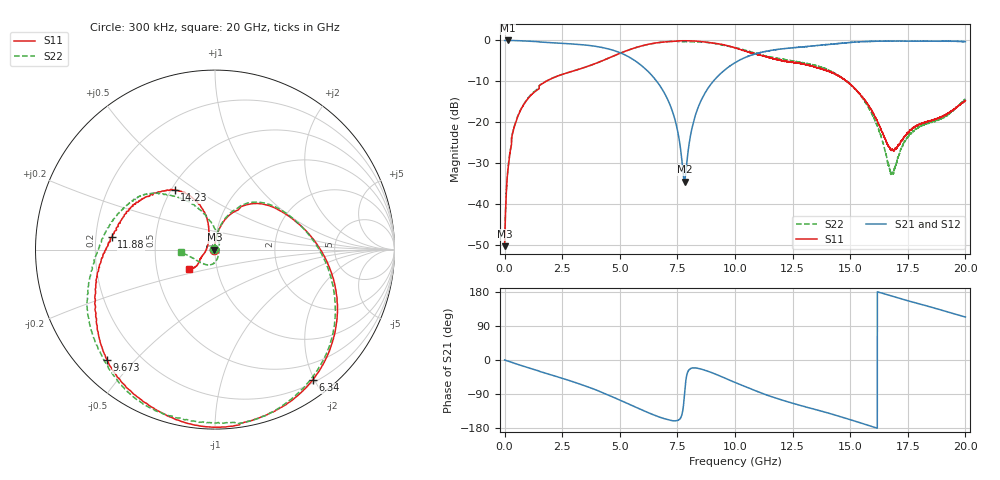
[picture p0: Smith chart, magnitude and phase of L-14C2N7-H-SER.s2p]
!{L-14C2N7}
!Johanson Technology Inc.
!www.johansontechnology.com
!Test Board Conditions:
!Substrate Type  RO4350B
!Substrate Thickness  20 mil
!Substrate Dk  3.66
!TL Type: GCPW
!TL Trace Width  36 mil
!TL Gap  12 mil
!Electrode orientation  Horizontal
!DUT TOPOLOGY	SERIES
!Mounting Pad LxW  26x36 mil
! Created Sun Jun 20 12:55:36 2021
# hz S ma R 50
! 2 Port Network Data from SP1.SP block
! freq  magS11  angS11  magS21  angS21  magS12  angS12  magS22  angS22
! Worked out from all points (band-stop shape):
!   20001 points, 300 kHz to 20 GHz, reference 50 ohm
!   highest |S21| = -0.02 dB at 130.3 MHz (marker M1); lowest = -34.6 dB at 7.81 GHz (marker M2)
!   |S21| within 3 dB of the highest: start of sweep to 5.007 GHz; 11.08 GHz to end of sweep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
!   lowest |S11| = -50.4 dB at 300 kHz (marker M3), VSWR 1.01, Z = 49.7 + j0.0289 ohm
!   |S11| at or under -10 dB: start of sweep to 1.807 GHz; 1.807622 GHz to 1.808451 GHz (828.7 kHz wide, 0.0458 % of centre); 14.85 GHz to end of sweep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
!   |S22| runs from -50.1 to -0.2 dB; largest |S21 - S12| = 0.016
!   S11 on the Smith chart (normalised r, x): 300 kHz: 0.99, +0.00; 6.34 GHz: 0.24, -1.97; 9.673 GHz: 0.09, -0.42; 11.88 GHz: 0.27, +0.06; 14.23 GHz: 0.52, +0.41; 20 GHz: 0.73, -0.17
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300000  0.003034 174.5  0.9973 -0.0  0.9966 -0.0  0.003125 169.6
1.303e8  0.02383 92.3  0.9979 -2.6  0.997 -2.5  0.02432 92.9
4.003e8  0.08329 82.4  0.9953 -8.2  0.995 -8.2  0.08482 82.7
8.923e8  0.1742 71.7  0.982 -17.8  0.9838 -17.9  0.1767 72.6
3.3343e9  0.4535 23.9  0.8859 -65.0  0.8859 -64.9  0.4541 24.9
4.6683e9  0.633 -7.0  0.7625 -96.8  0.7631 -96.7  0.633 -8.6
6.3403e9  0.9082 -53.2  0.3861 -141.6  0.3867 -141.3  0.9028 -54.7
6.6673e9  0.9393 -61.8  0.2982 -149.4  0.2976 -149.1  0.9358 -63.4
7.3613e9  0.9753 -78.9  0.1153 -160.5  0.1157 -160.5  0.9758 -79.9
7.8103e9  0.99 -88.6  0.01866 -88.2  0.0188 -87.7  0.9651 -91.5
8.1223e9  0.9862 -95.1  0.08152 -21.5  0.08207 -20.8  0.9608 -99.6
8.4343e9  0.973 -102.2  0.1601 -22.6  0.16 -22.1  0.9576 -107.8
9.6733e9  0.8604 -134.3  0.4618 -50.7  0.4673 -50.7  0.8525 -139.9
1.00003e10  0.8116 -142.6  0.5336 -59.2  0.5361 -59.1  0.8147 -148.7
1.18763e10  0.5793 173.2  0.7766 -102.6  0.7775 -102.9  0.6018 166.5
1.33343e10  0.4848 142.8  0.8536 -128.2  0.8481 -128.4  0.5065 143.5
1.42333e10  0.4022 124.1  0.9009 -143.4  0.8947 -143.6  0.4065 131.3
1.57133e10  0.1718 104.3  0.9679 -171.1  0.9657 -171.1  0.1648 100.5
1.66673e10  0.05052 139.1  0.9817 171.0  0.9817 171.1  0.02944 35.0
1.68483e10  0.04589 162.0  0.9818 167.7  0.9815 167.9  0.02395 -13.8
1.77483e10  0.08587 -151.3  0.9783 152.3  0.9745 152.2  0.07698 -95.7
2e10  0.1833 -143.2  0.9649 113.4  0.9583 113.1  0.1927 -176.4
